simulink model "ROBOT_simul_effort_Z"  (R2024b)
settings: Solver=VariableStepAuto  StartTime=0.0  StopTime=5  RelTol=1e-3
undefined symbols (not defined in the file): a, ARRIERE_Defaut_sldprt, avant01_Defaut_sldprt, avant02_Defaut_sldprt, avant03_Defaut_sldprt, avant1_Defaut_sldprt, AXE, BASE_Defaut_sldprt, BIELLE, BIELLE_Defaut_sldprt, BRAS_Defaut_sldprt, bras_Defaut_sldprt, C_Realiste_sldprt, CABLE_Defaut_sldprt, cable_Defaut_sldprt, CACHE_Defaut_sldprt, CARTE, carte_Defaut_sldprt, CARTER, carter, CHC, CODEUR_Defaut_sldprt, cruciforme, cylindrique, deg, Drive, Fichiers, Fichiers_Matlab_sujetA, FIXATION, fixation_Defaut_sldprt, H, HEXAGONALE_Defaut_sldprt, joint_Defaut_sldprt, kg, m, M4, M4_Defaut_sldprt, manette1_Defaut_sldprt, manette2_Defaut_sldprt, MATLAB, Matlab, matlab_Defaut_sldprt, mm, modif, MOTEUR_Defaut_sldprt, N, NEZ_Defaut_sldprt, nom, palier, PARALLELOGRAMME_Defaut_sldprt, petite, plaque, rad, Ressort, Rondelle, ROTOR_Defaut_sldprt, s, SET, simple, socle_Defaut_sldprt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
libraries: sm_lib x463, fl_lib x45, nesl_utility x27, simulink x2
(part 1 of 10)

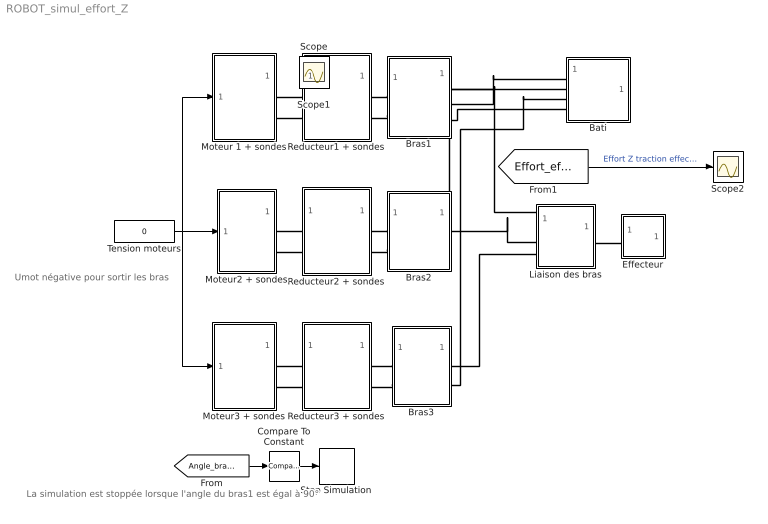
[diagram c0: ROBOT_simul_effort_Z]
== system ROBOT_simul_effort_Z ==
  note: La simulation est stoppée lorsque l'angle du bras1 est égal à 90°
  note: Umot négative pour sortir les bras
  Bati : Subsystem
  Bras1 : Subsystem
  Bras2 : Subsystem
  Bras3 : Subsystem
  Compare To Constant : simulink/Logic and Bit Operations/Compare To Constant  relop=>=  const=85  OutDataTypeStr=boolean
  Effecteur : Subsystem
  Liaison des bras : Subsystem
  Moteur 1 + sondes : Subsystem
  Moteur2 + sondes : Subsystem
  Moteur3 + sondes : Subsystem
  Reducteur1 + sondes : Subsystem
  Reducteur2 + sondes : Subsystem
  Reducteur3 + sondes : Subsystem
  Scope2 : Scope
  Stop Simulation : Stop
  Tension moteurs : Constant  Value=0
  Scope : Scope
  Scope1 : Scope
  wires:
  [Angle_bras1] -> Compare To Constant/1
  Compare To Constant/1 -> Stop Simulation/1
  Tension moteurs/1 -> Moteur2 + sondes/1(In1), Moteur 1 + sondes/1(In1), Moteur3 + sondes/1(In1)
  [Effort_effecteur] -> Scope2/1  "Effort Z traction effecteur (N)"
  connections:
  Bras3/RConn2 -- Bati/LConn3
  Bras1/LConn2 -- Reducteur1 + sondes/RConn2
  Bras2/RConn2 -- Bati/LConn2
  Moteur3 + sondes/RConn2 -- Reducteur3 + sondes/LConn2
  Bras1/RConn2 -- Bati/LConn1
  Bras1/RConn3 -- Bati/LConn4
  Liaison des bras/LConn1 -- Bras1/RConn1
  Bras3/LConn1 -- Reducteur3 + sondes/RConn1
  Moteur 1 + sondes/RConn1 -- Reducteur1 + sondes/LConn1
  Liaison des bras/LConn3 -- Bras3/RConn1
  Liaison des bras/RConn1 -- Effecteur/LConn1
  Liaison des bras/LConn2 -- Bras2/RConn1
  Moteur2 + sondes/RConn1 -- Reducteur2 + sondes/LConn1
  Bras1/LConn1 -- Reducteur1 + sondes/RConn1
  Bras3/LConn2 -- Reducteur3 + sondes/RConn2
  Moteur2 + sondes/RConn2 -- Reducteur2 + sondes/LConn2
  Bras2/LConn2 -- Reducteur2 + sondes/RConn2
  Moteur 1 + sondes/RConn2 -- Reducteur1 + sondes/LConn2
  Bras2/LConn1 -- Reducteur2 + sondes/RConn1
  Moteur3 + sondes/RConn1 -- Reducteur3 + sondes/LConn1

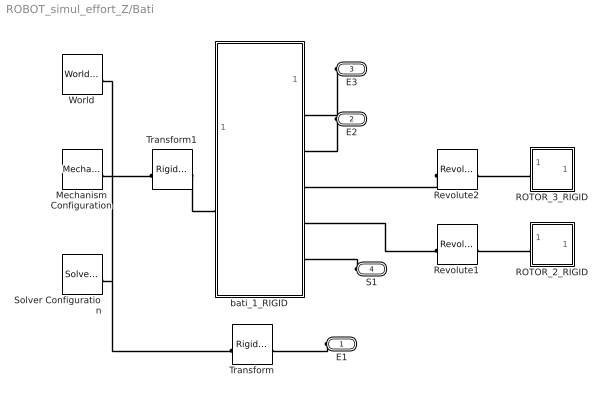
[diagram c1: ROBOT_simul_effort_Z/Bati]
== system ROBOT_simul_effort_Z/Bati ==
  Mechanism Configuration : sm_lib/Utilities/Mechanism Configuration  UniformGravity=Constant  GravityVector=[0 -9.81 0]  GravityVectorUnits=m/s^2  LinearizationDelta=0.001  JointModeTransitionNonlinearIterations=2
  ROTOR_2_RIGID : Subsystem
  ROTOR_3_RIGID : Subsystem
  Revolute1 : sm_lib/Joints/Revolute Joint  JointMode=Normal  CompositeWrenchDir=FollowerOnBase  CompositeWrenchFrame=BaseFrame  SenseConstraintForce=off  SenseConstraintTorque=off  SenseTotalForce=off  SenseTotalTorque=off  PositionTargetSpecify=on  PositionTargetPriority=Low  PositionTargetValue=-26.406351854743253  PositionTargetValueUnits=deg  VelocityTargetSpecify=off  VelocityTargetPriority=High  VelocityTargetValue=0  VelocityTargetValueUnits=deg/s  EquilibriumPosition=0  EquilibriumPositionUnits=rad  SpringStiffness=0  SpringStiffnessUnits=m*N/rad  DampingCoefficient=0  DampingCoefficientUnits=m*s*N/rad  LowerLimitSpecify=off  LowerLimitBound=-90  LowerLimitBoundUnits=deg  LowerLimitStiffness=1e4  LowerLimitStiffnessUnits=N*m/deg  LowerLimitDamping=10  LowerLimitDampingUnits=N*m/(deg/s)  LowerLimitTransitionRegionWidth=0.1  LowerLimitTransitionRegionWidthUnits=deg  UpperLimitSpecify=off  UpperLimitBound=90  UpperLimitBoundUnits=deg  UpperLimitStiffness=1e4  UpperLimitStiffnessUnits=N*m/deg  UpperLimitDamping=10  UpperLimitDampingUnits=N*m/(deg/s)  UpperLimitTransitionRegionWidth=0.1  UpperLimitTransitionRegionWidthUnits=deg  TorqueActuationMode=NoTorque  MotionActuationMode=ComputedMotion  SensePosition=off  SenseVelocity=off  SenseAcceleration=off  SenseTorqueForce=off  SenseLowerLimitTorqueForce=off  SenseUpperLimitTorqueForce=off
  Revolute2 : sm_lib/Joints/Revolute Joint  JointMode=Normal  CompositeWrenchDir=FollowerOnBase  CompositeWrenchFrame=BaseFrame  SenseConstraintForce=off  SenseConstraintTorque=off  SenseTotalForce=off  SenseTotalTorque=off  PositionTargetSpecify=on  PositionTargetPriority=Low  PositionTargetValue=-61.713604489421797  PositionTargetValueUnits=deg  VelocityTargetSpecify=off  VelocityTargetPriority=High  VelocityTargetValue=0  VelocityTargetValueUnits=deg/s  EquilibriumPosition=0  EquilibriumPositionUnits=rad  SpringStiffness=0  SpringStiffnessUnits=m*N/rad  DampingCoefficient=0  DampingCoefficientUnits=m*s*N/rad  LowerLimitSpecify=off  LowerLimitBound=-90  LowerLimitBoundUnits=deg  LowerLimitStiffness=1e4  LowerLimitStiffnessUnits=N*m/deg  LowerLimitDamping=10  LowerLimitDampingUnits=N*m/(deg/s)  LowerLimitTransitionRegionWidth=0.1  LowerLimitTransitionRegionWidthUnits=deg  UpperLimitSpecify=off  UpperLimitBound=90  UpperLimitBoundUnits=deg  UpperLimitStiffness=1e4  UpperLimitStiffnessUnits=N*m/deg  UpperLimitDamping=10  UpperLimitDampingUnits=N*m/(deg/s)  UpperLimitTransitionRegionWidth=0.1  UpperLimitTransitionRegionWidthUnits=deg  TorqueActuationMode=NoTorque  MotionActuationMode=ComputedMotion  SensePosition=off  SenseVelocity=off  SenseAcceleration=off  SenseTorqueForce=off  SenseLowerLimitTorqueForce=off  SenseUpperLimitTorqueForce=off
  Solver Configuration : nesl_utility/Solver Configuration  PhysicalDomain=network_engine_domain  SubClassName=solver  LeftPortType=input  RightPortType=generic  Tones=[]  Harmonics=[]  SimulateNoise=off  Profile=off  UseLocalSampling=off  EnableSwitchedLinearOptims=on  FrequencyDomain=off  UseCCode=off  RelTol=0.001  AbsTol=1e-06  MinStep=1e-09  ToWorkspace=off  RevertToSquareIcSolve=off  NumHomotopyIterations=100  PhasorMode=off  PhasorModeNumHarmonics=1  ConsistencySolver=NEWTON_FTOL  IndexReductionMethod=DerivativeReplacement  DoDC=off  ResidualTolerance=1e-09  ConsistencyTolSource=GLOBAL  ConsistencyAbsTol=0.001  ConsistencyRelTol=0.001  ConsistencyTolFactor=0.001  UseLocalSolver=off  LocalSolverChoice=NE_BACKWARD_EULER_ADVANCER  ResolveIndetEquations=on  FunctionEvalNumThread=1  LocalSolverSampleTime=0.001  DoFixedCost=off  MaxNonlinIter=3  MaxModeIter=2  ComputeImpulses=off  ImpulseIterations=2  LinearAlgebra=Sparse  LinearAlgebraNumThread=0  EquationFormulation=NE_TIME_EF  DelaysMemoryBudget=1024  AutomaticFiltering=on  FilteringTimeConstant=0.001  PartitionStorageMethod=AS_NEEDED  PartitionMemoryBudget=1024  PartitionMethod=FAST  MultibodyUseLocalSolver=off  MultibodyLocalSolverChoice=ODE1  MultibodyLocalSolverSampleTime=0.001
  Transform : sm_lib/Frames and Transforms/Rigid Transform  RotationMethod=ArbitraryAxis  FollAlignAxisA=+X  BaseAlignAxisA=+Y  FollAlignAxisB=+Y  BaseAlignAxisB=+Z  RotationStandardAxis=+Z  RotationAngle=2.2576709855630148  RotationAngleUnits=rad  RotationArbitraryAxis=[0.47317816576135285 0.62293756647304621 0.6229375664730461]  RotationSequenceAxes=FollowerAxes  RotationSequence=XYX  RotationSequenceAngles=[0 0 0]  RotationSequenceAnglesUnits=deg  RotationMatrix=[1 0 0; 0 1 0; 0 0 1]  Quaternion=[1 0 0 0]  TranslationMethod=Cartesian  TranslationCartesianOffset=[-50.295220189469383 24.641508789034031 0]  TranslationCartesianOffsetUnits=mm  TranslationStandardAxis=+Z  TranslationStandardOffset=0  TranslationStandardOffsetUnits=mm  TranslationROffset=0  TranslationROffsetUnits=m  TranslationThetaOffset=0  TranslationThetaOffsetUnits=deg  TranslationZOffset=0  TranslationZOffsetUnits=m
  Transform1 : sm_lib/Frames and Transforms/Rigid Transform  RotationMethod=None  FollAlignAxisA=+X  BaseAlignAxisA=+Y  FollAlignAxisB=+Y  BaseAlignAxisB=+Z  RotationStandardAxis=+Z  RotationAngle=0  RotationAngleUnits=deg  RotationArbitraryAxis=[0 0 1]  RotationSequenceAxes=FollowerAxes  RotationSequence=XYX  RotationSequenceAngles=[0 0 0]  RotationSequenceAnglesUnits=deg  RotationMatrix=[1 0 0; 0 1 0; 0 0 1]  Quaternion=[1 0 0 0]  TranslationMethod=Cartesian  TranslationCartesianOffset=[0 -115.25004756062962 -99.318100969999989]  TranslationCartesianOffsetUnits=mm  TranslationStandardAxis=+Z  TranslationStandardOffset=0  TranslationStandardOffsetUnits=mm  TranslationROffset=0  TranslationROffsetUnits=m  TranslationThetaOffset=0  TranslationThetaOffsetUnits=deg  TranslationZOffset=0  TranslationZOffsetUnits=m
  World : sm_lib/Frames and Transforms/World Frame
  bati_1_RIGID : Subsystem
  E1 : PMIOPort  Side=Left
  E2 : PMIOPort  Port=2  Side=Left
  E3 : PMIOPort  Port=3  Side=Left
  S1 : PMIOPort  Port=4  Side=Left
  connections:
  Mechanism Configuration/RConn1 -- Transform/LConn1 -- Solver Configuration/RConn1 -- World/RConn1 -- Transform1/LConn1
  ROTOR_3_RIGID/LConn1 -- Revolute2/RConn1
  Transform1/RConn1 -- bati_1_RIGID/LConn1
  Revolute2/LConn1 -- bati_1_RIGID/RConn3
  E2/RConn1 -- bati_1_RIGID/RConn2
  E1/RConn1 -- Transform/RConn1
  E3/RConn1 -- bati_1_RIGID/RConn1
  ROTOR_2_RIGID/LConn1 -- Revolute1/RConn1
  S1/RConn1 -- bati_1_RIGID/RConn5
  Revolute1/LConn1 -- bati_1_RIGID/RConn4

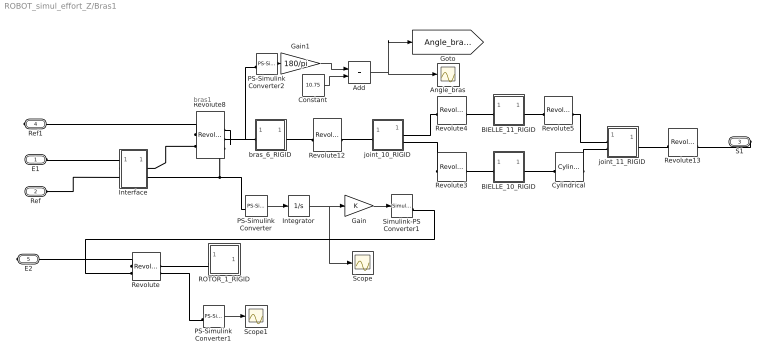
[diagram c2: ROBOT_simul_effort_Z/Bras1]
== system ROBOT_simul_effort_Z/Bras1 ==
  note: bras1
  Add : Sum
  Angle_bras : Scope
  BIELLE_10_RIGID : Subsystem
  BIELLE_11_RIGID : Subsystem
  Constant : Constant  Value=10.75
  Cylindrical : sm_lib/Joints/Cylindrical Joint  JointMode=Normal  CompositeWrenchDir=FollowerOnBase  CompositeWrenchFrame=BaseFrame  SenseConstraintForce=off  SenseConstraintTorque=off  SenseTotalForce=off  SenseTotalTorque=off  RzPositionTargetSpecify=off  RzPositionTargetPriority=High  RzPositionTargetValue=0  RzPositionTargetValueUnits=deg  RzVelocityTargetSpecify=off  RzVelocityTargetPriority=High  RzVelocityTargetValue=0  RzVelocityTargetValueUnits=deg/s  RzEquilibriumPosition=0  RzEquilibriumPositionUnits=rad  RzSpringStiffness=0  RzSpringStiffnessUnits=m*N/rad  RzDampingCoefficient=0  RzDampingCoefficientUnits=m*s*N/rad  RzLowerLimitSpecify=off  RzLowerLimitBound=-90  RzLowerLimitBoundUnits=deg  RzLowerLimitStiffness=1e4  RzLowerLimitStiffnessUnits=N*m/deg  RzLowerLimitDamping=10  RzLowerLimitDampingUnits=N*m/(deg/s)  RzLowerLimitTransitionRegionWidth=0.1  RzLowerLimitTransitionRegionWidthUnits=deg  RzUpperLimitSpecify=off  RzUpperLimitBound=90  RzUpperLimitBoundUnits=deg  RzUpperLimitStiffness=1e4  RzUpperLimitStiffnessUnits=N*m/deg  RzUpperLimitDamping=10  RzUpperLimitDampingUnits=N*m/(deg/s)  RzUpperLimitTransitionRegionWidth=0.1  RzUpperLimitTransitionRegionWidthUnits=deg  RzTorqueActuationMode=NoTorque  RzMotionActuationMode=ComputedMotion  RzSensePosition=off  RzSenseVelocity=off  RzSenseAcceleration=off  RzSenseTorqueForce=off  RzSenseLowerLimitTorqueForce=off  RzSenseUpperLimitTorqueForce=off  PzPositionTargetSpecify=off  PzPositionTargetPriority=High  PzPositionTargetValue=0  PzPositionTargetValueUnits=m  PzVelocityTargetSpecify=off  PzVelocityTargetPriority=High  PzVelocityTargetValue=0  PzVelocityTargetValueUnits=m/s  PzEquilibriumPosition=0  PzEquilibriumPositionUnits=m  PzSpringStiffness=0  PzSpringStiffnessUnits=N/m  PzDampingCoefficient=0  PzDampingCoefficientUnits=s*N/m  PzLowerLimitSpecify=off  PzLowerLimitBound=-1  PzLowerLimitBoundUnits=m  PzLowerLimitStiffness=1e6  PzLowerLimitStiffnessUnits=N/m  PzLowerLimitDamping=1e3  PzLowerLimitDampingUnits=N/(m/s)  PzLowerLimitTransitionRegionWidth=1e-4  PzLowerLimitTransitionRegionWidthUnits=m  PzUpperLimitSpecify=off  PzUpperLimitBound=1  PzUpperLimitBoundUnits=m  PzUpperLimitStiffness=1e6  PzUpperLimitStiffnessUnits=N/m  PzUpperLimitDamping=1e3  PzUpperLimitDampingUnits=N/(m/s)  PzUpperLimitTransitionRegionWidth=1e-4  PzUpperLimitTransitionRegionWidthUnits=m  PzTorqueActuationMode=NoTorque  PzMotionActuationMode=ComputedMotion  PzSensePosition=off  PzSenseVelocity=off  PzSenseAcceleration=off  PzSenseTorqueForce=off  PzSenseLowerLimitTorqueForce=off  PzSenseUpperLimitTorqueForce=off
  Gain : Gain
  Gain1 : Gain  Gain=180/pi
  Integrator : Integrator
  Interface : Subsystem
  PS-Simulink Converter : nesl_utility/PS-Simulink Converter  PhysicalDomain=network_engine_domain  SubClassName=ps_output  LeftPortType=input  RightPortType=output  PseudoPeriodic=off  Frequencies=[]  VectorFormat=1-D array  Unit=1  AffineConversion=off
  PS-Simulink Converter1 : nesl_utility/PS-Simulink Converter  PhysicalDomain=network_engine_domain  SubClassName=ps_output  LeftPortType=input  RightPortType=output  PseudoPeriodic=off  Frequencies=[]  VectorFormat=1-D array  Unit=1  AffineConversion=off
  PS-Simulink Converter2 : nesl_utility/PS-Simulink Converter  PhysicalDomain=network_engine_domain  SubClassName=ps_output  LeftPortType=input  RightPortType=output  PseudoPeriodic=off  Frequencies=[]  VectorFormat=1-D array  Unit=1  AffineConversion=off
  ROTOR_1_RIGID : Subsystem
  Revolute : sm_lib/Joints/Revolute Joint  JointMode=Normal  CompositeWrenchDir=FollowerOnBase  CompositeWrenchFrame=BaseFrame  SenseConstraintForce=off  SenseConstraintTorque=off  SenseTotalForce=off  SenseTotalTorque=off  PositionTargetSpecify=on  PositionTargetPriority=Low  PositionTargetValue=-79.560971310790379  PositionTargetValueUnits=deg  VelocityTargetSpecify=off  VelocityTargetPriority=High  VelocityTargetValue=0  VelocityTargetValueUnits=deg/s  EquilibriumPosition=0  EquilibriumPositionUnits=rad  SpringStiffness=0  SpringStiffnessUnits=m*N/rad  DampingCoefficient=0  DampingCoefficientUnits=m*s*N/rad  LowerLimitSpecify=off  LowerLimitBound=-90  LowerLimitBoundUnits=deg  LowerLimitStiffness=1e4  LowerLimitStiffnessUnits=N*m/deg  LowerLimitDamping=10  LowerLimitDampingUnits=N*m/(deg/s)  LowerLimitTransitionRegionWidth=0.1  LowerLimitTransitionRegionWidthUnits=deg  UpperLimitSpecify=off  UpperLimitBound=90  UpperLimitBoundUnits=deg  UpperLimitStiffness=1e4  UpperLimitStiffnessUnits=N*m/deg  UpperLimitDamping=10  UpperLimitDampingUnits=N*m/(deg/s)  UpperLimitTransitionRegionWidth=0.1  UpperLimitTransitionRegionWidthUnits=deg  TorqueActuationMode=ComputedTorque  MotionActuationMode=InputMotion  SensePosition=off  SenseVelocity=on  SenseAcceleration=off  SenseTorqueForce=off  SenseLowerLimitTorqueForce=off  SenseUpperLimitTorqueForce=off
  Revolute12 : sm_lib/Joints/Revolute Joint  JointMode=Normal  CompositeWrenchDir=FollowerOnBase  CompositeWrenchFrame=BaseFrame  SenseConstraintForce=off  SenseConstraintTorque=off  SenseTotalForce=off  SenseTotalTorque=off  PositionTargetSpecify=on  PositionTargetPriority=Low  PositionTargetValue=114.87234196171698  PositionTargetValueUnits=deg  VelocityTargetSpecify=off  VelocityTargetPriority=High  VelocityTargetValue=0  VelocityTargetValueUnits=deg/s  EquilibriumPosition=0  EquilibriumPositionUnits=rad  SpringStiffness=0  SpringStiffnessUnits=m*N/rad  DampingCoefficient=0  DampingCoefficientUnits=m*s*N/rad  LowerLimitSpecify=off  LowerLimitBound=-90  LowerLimitBoundUnits=deg  LowerLimitStiffness=1e4  LowerLimitStiffnessUnits=N*m/deg  LowerLimitDamping=10  LowerLimitDampingUnits=N*m/(deg/s)  LowerLimitTransitionRegionWidth=0.1  LowerLimitTransitionRegionWidthUnits=deg  UpperLimitSpecify=off  UpperLimitBound=90  UpperLimitBoundUnits=deg  UpperLimitStiffness=1e4  UpperLimitStiffnessUnits=N*m/deg  UpperLimitDamping=10  UpperLimitDampingUnits=N*m/(deg/s)  UpperLimitTransitionRegionWidth=0.1  UpperLimitTransitionRegionWidthUnits=deg  TorqueActuationMode=NoTorque  MotionActuationMode=ComputedMotion  SensePosition=off  SenseVelocity=off  SenseAcceleration=off  SenseTorqueForce=off  SenseLowerLimitTorqueForce=off  SenseUpperLimitTorqueForce=off
  Revolute13 : sm_lib/Joints/Revolute Joint  JointMode=Normal  CompositeWrenchDir=FollowerOnBase  CompositeWrenchFrame=BaseFrame  SenseConstraintForce=off  SenseConstraintTorque=off  SenseTotalForce=off  SenseTotalTorque=off  PositionTargetSpecify=off  PositionTargetPriority=High  PositionTargetValue=0  PositionTargetValueUnits=deg  VelocityTargetSpecify=off  VelocityTargetPriority=High  VelocityTargetValue=0  VelocityTargetValueUnits=deg/s  EquilibriumPosition=0  EquilibriumPositionUnits=rad  SpringStiffness=0  SpringStiffnessUnits=m*N/rad  DampingCoefficient=0  DampingCoefficientUnits=m*s*N/rad  LowerLimitSpecify=off  LowerLimitBound=-90  LowerLimitBoundUnits=deg  LowerLimitStiffness=1e4  LowerLimitStiffnessUnits=N*m/deg  LowerLimitDamping=10  LowerLimitDampingUnits=N*m/(deg/s)  LowerLimitTransitionRegionWidth=0.1  LowerLimitTransitionRegionWidthUnits=deg  UpperLimitSpecify=off  UpperLimitBound=90  UpperLimitBoundUnits=deg  UpperLimitStiffness=1e4  UpperLimitStiffnessUnits=N*m/deg  UpperLimitDamping=10  UpperLimitDampingUnits=N*m/(deg/s)  UpperLimitTransitionRegionWidth=0.1  UpperLimitTransitionRegionWidthUnits=deg  TorqueActuationMode=NoTorque  MotionActuationMode=ComputedMotion  SensePosition=off  SenseVelocity=off  SenseAcceleration=off  SenseTorqueForce=off  SenseLowerLimitTorqueForce=off  SenseUpperLimitTorqueForce=off
  Revolute3 : sm_lib/Joints/Revolute Joint  JointMode=Normal  CompositeWrenchDir=FollowerOnBase  CompositeWrenchFrame=BaseFrame  SenseConstraintForce=off  SenseConstraintTorque=off  SenseTotalForce=off  SenseTotalTorque=off  PositionTargetSpecify=on  PositionTargetPriority=Low  PositionTargetValue=-1.4448284825041595  PositionTargetValueUnits=deg  VelocityTargetSpecify=off  VelocityTargetPriority=High  VelocityTargetValue=0  VelocityTargetValueUnits=deg/s  EquilibriumPosition=0  EquilibriumPositionUnits=rad  SpringStiffness=0  SpringStiffnessUnits=m*N/rad  DampingCoefficient=0  DampingCoefficientUnits=m*s*N/rad  LowerLimitSpecify=off  LowerLimitBound=-90  LowerLimitBoundUnits=deg  LowerLimitStiffness=1e4  LowerLimitStiffnessUnits=N*m/deg  LowerLimitDamping=10  LowerLimitDampingUnits=N*m/(deg/s)  LowerLimitTransitionRegionWidth=0.1  LowerLimitTransitionRegionWidthUnits=deg  UpperLimitSpecify=off  UpperLimitBound=90  UpperLimitBoundUnits=deg  UpperLimitStiffness=1e4  UpperLimitStiffnessUnits=N*m/deg  UpperLimitDamping=10  UpperLimitDampingUnits=N*m/(deg/s)  UpperLimitTransitionRegionWidth=0.1  UpperLimitTransitionRegionWidthUnits=deg  TorqueActuationMode=NoTorque  MotionActuationMode=ComputedMotion  SensePosition=off  SenseVelocity=off  SenseAcceleration=off  SenseTorqueForce=off  SenseLowerLimitTorqueForce=off  SenseUpperLimitTorqueForce=off
  Revolute4 : sm_lib/Joints/Revolute Joint  JointMode=Normal  CompositeWrenchDir=FollowerOnBase  CompositeWrenchFrame=BaseFrame  SenseConstraintForce=off  SenseConstraintTorque=off  SenseTotalForce=off  SenseTotalTorque=off  PositionTargetSpecify=on  PositionTargetPriority=Low  PositionTargetValue=1.4448284825041535  PositionTargetValueUnits=deg  VelocityTargetSpecify=off  VelocityTargetPriority=High  VelocityTargetValue=0  VelocityTargetValueUnits=deg/s  EquilibriumPosition=0  EquilibriumPositionUnits=rad  SpringStiffness=0  SpringStiffnessUnits=m*N/rad  DampingCoefficient=0  DampingCoefficientUnits=m*s*N/rad  LowerLimitSpecify=off  LowerLimitBound=-90  LowerLimitBoundUnits=deg  LowerLimitStiffness=1e4  LowerLimitStiffnessUnits=N*m/deg  LowerLimitDamping=10  LowerLimitDampingUnits=N*m/(deg/s)  LowerLimitTransitionRegionWidth=0.1  LowerLimitTransitionRegionWidthUnits=deg  UpperLimitSpecify=off  UpperLimitBound=90  UpperLimitBoundUnits=deg  UpperLimitStiffness=1e4  UpperLimitStiffnessUnits=N*m/deg  UpperLimitDamping=10  UpperLimitDampingUnits=N*m/(deg/s)  UpperLimitTransitionRegionWidth=0.1  UpperLimitTransitionRegionWidthUnits=deg  TorqueActuationMode=NoTorque  MotionActuationMode=ComputedMotion  SensePosition=off  SenseVelocity=off  SenseAcceleration=off  SenseTorqueForce=off  SenseLowerLimitTorqueForce=off  SenseUpperLimitTorqueForce=off
  Revolute5 : sm_lib/Joints/Revolute Joint  JointMode=Normal  CompositeWrenchDir=FollowerOnBase  CompositeWrenchFrame=BaseFrame  SenseConstraintForce=off  SenseConstraintTorque=off  SenseTotalForce=off  SenseTotalTorque=off  PositionTargetSpecify=on  PositionTargetPriority=Low  PositionTargetValue=-178.55517151749589  PositionTargetValueUnits=deg  VelocityTargetSpecify=off  VelocityTargetPriority=High  VelocityTargetValue=0  VelocityTargetValueUnits=deg/s  EquilibriumPosition=0  EquilibriumPositionUnits=rad  SpringStiffness=0  SpringStiffnessUnits=m*N/rad  DampingCoefficient=0  DampingCoefficientUnits=m*s*N/rad  LowerLimitSpecify=off  LowerLimitBound=-90  LowerLimitBoundUnits=deg  LowerLimitStiffness=1e4  LowerLimitStiffnessUnits=N*m/deg  LowerLimitDamping=10  LowerLimitDampingUnits=N*m/(deg/s)  LowerLimitTransitionRegionWidth=0.1  LowerLimitTransitionRegionWidthUnits=deg  UpperLimitSpecify=off  UpperLimitBound=90  UpperLimitBoundUnits=deg  UpperLimitStiffness=1e4  UpperLimitStiffnessUnits=N*m/deg  UpperLimitDamping=10  UpperLimitDampingUnits=N*m/(deg/s)  UpperLimitTransitionRegionWidth=0.1  UpperLimitTransitionRegionWidthUnits=deg  TorqueActuationMode=NoTorque  MotionActuationMode=ComputedMotion  SensePosition=off  SenseVelocity=off  SenseAcceleration=off  SenseTorqueForce=off  SenseLowerLimitTorqueForce=off  SenseUpperLimitTorqueForce=off
  Revolute8 : sm_lib/Joints/Revolute Joint  JointMode=Normal  CompositeWrenchDir=FollowerOnBase  CompositeWrenchFrame=BaseFrame  SenseConstraintForce=off  SenseConstraintTorque=off  SenseTotalForce=off  SenseTotalTorque=off  PositionTargetSpecify=on  PositionTargetPriority=Low  PositionTargetValue=-11.877849818911594  PositionTargetValueUnits=deg  VelocityTargetSpecify=off  VelocityTargetPriority=High  VelocityTargetValue=0  VelocityTargetValueUnits=deg/s  EquilibriumPosition=0  EquilibriumPositionUnits=rad  SpringStiffness=0  SpringStiffnessUnits=m*N/rad  DampingCoefficient=0  DampingCoefficientUnits=m*s*N/rad  LowerLimitSpecify=off  LowerLimitBound=-90  LowerLimitBoundUnits=deg  LowerLimitStiffness=1e4  LowerLimitStiffnessUnits=N*m/deg  LowerLimitDamping=10  LowerLimitDampingUnits=N*m/(deg/s)  LowerLimitTransitionRegionWidth=0.1  LowerLimitTransitionRegionWidthUnits=deg  UpperLimitSpecify=off  UpperLimitBound=90  UpperLimitBoundUnits=deg  UpperLimitStiffness=1e4  UpperLimitStiffnessUnits=N*m/deg  UpperLimitDamping=10  UpperLimitDampingUnits=N*m/(deg/s)  UpperLimitTransitionRegionWidth=0.1  UpperLimitTransitionRegionWidthUnits=deg  TorqueActuationMode=InputTorque  MotionActuationMode=ComputedMotion  SensePosition=on  SenseVelocity=on  SenseAcceleration=off  SenseTorqueForce=off  SenseLowerLimitTorqueForce=off  SenseUpperLimitTorqueForce=off
  Scope : Scope
  Scope1 : Scope
  Simulink-PS Converter1 : nesl_utility/Simulink-PS Converter  PhysicalDomain=network_engine_domain  SubClassName=ps_input  LeftPortType=input  RightPortType=output  PseudoPeriodic=off  Frequencies=[]  NoiseDistribution=none  NoiseParameters=[]  Unit=1  AffineConversion=off  FilteringAndDerivatives=filter  SimscapeFilterOrder=2  InputFilterTimeConstant=1e-4  UdotUserProvided=1
  bras_6_RIGID : Subsystem
  joint_10_RIGID : Subsystem
  joint_11_RIGID : Subsystem
  E1 : PMIOPort  Side=Left
  Ref : PMIOPort  Port=2  Side=Left
  S1 : PMIOPort  Port=3  Side=Right
  Ref1 : PMIOPort  Port=4  Side=Right
  E2 : PMIOPort  Port=5  Side=Right
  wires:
  PS-Simulink Converter/1 -> Integrator/1
  Gain/1 -> Simulink-PS Converter1/1
  PS-Simulink Converter1/1 -> Scope1/1
  Integrator/1 -> Scope/1, Gain/1
  PS-Simulink Converter2/1 -> Gain1/1
  Gain1/1 -> Add/1
  Add/1 -> Angle_bras/1, [Angle_bras1]
  Constant/1 -> Add/2
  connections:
  Interface/RConn1 -- Revolute8/LConn2
  Interface/RConn2 -- Revolute8/RConn3 -- PS-Simulink Converter/LConn1
  Ref/RConn1 -- Interface/LConn2
  Interface/LConn1 -- E1/RConn1
  BIELLE_11_RIGID/LConn1 -- Revolute4/LConn1
  BIELLE_10_RIGID/RConn1 -- Cylindrical/LConn1
  Revolute4/RConn1 -- joint_10_RIGID/RConn1
  Cylindrical/RConn1 -- joint_11_RIGID/LConn2
  BIELLE_11_RIGID/RConn1 -- Revolute5/LConn1
  Revolute12/LConn1 -- bras_6_RIGID/RConn1
  Revolute12/RConn1 -- joint_10_RIGID/LConn1
  Revolute8/RConn1 -- bras_6_RIGID/LConn1
  Revolute8/LConn1 -- Ref1/RConn1
  Revolute5/RConn1 -- joint_11_RIGID/LConn1
  Revolute13/RConn1 -- joint_11_RIGID/RConn1
  S1/RConn1 -- Revolute13/LConn1
  Revolute3/RConn1 -- joint_10_RIGID/RConn2
  BIELLE_10_RIGID/LConn1 -- Revolute3/LConn1
  ROTOR_1_RIGID/LConn1 -- Revolute/RConn1
  Revolute/LConn1 -- E2/RConn1
  Revolute/LConn2 -- Simulink-PS Converter1/RConn1
  PS-Simulink Converter1/LConn1 -- Revolute/RConn2
  PS-Simulink Converter2/LConn1 -- Revolute8/RConn2

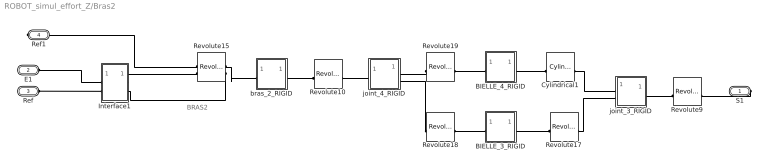
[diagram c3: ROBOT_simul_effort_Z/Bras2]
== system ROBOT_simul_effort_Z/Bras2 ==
  note: BRAS2
  BIELLE_3_RIGID : Subsystem
  BIELLE_4_RIGID : Subsystem
  Cylindrical1 : sm_lib/Joints/Cylindrical Joint  JointMode=Normal  CompositeWrenchDir=FollowerOnBase  CompositeWrenchFrame=BaseFrame  SenseConstraintForce=off  SenseConstraintTorque=off  SenseTotalForce=off  SenseTotalTorque=off  RzPositionTargetSpecify=off  RzPositionTargetPriority=High  RzPositionTargetValue=0  RzPositionTargetValueUnits=deg  RzVelocityTargetSpecify=off  RzVelocityTargetPriority=High  RzVelocityTargetValue=0  RzVelocityTargetValueUnits=deg/s  RzEquilibriumPosition=0  RzEquilibriumPositionUnits=rad  RzSpringStiffness=0  RzSpringStiffnessUnits=m*N/rad  RzDampingCoefficient=0  RzDampingCoefficientUnits=m*s*N/rad  RzLowerLimitSpecify=off  RzLowerLimitBound=-90  RzLowerLimitBoundUnits=deg  RzLowerLimitStiffness=1e4  RzLowerLimitStiffnessUnits=N*m/deg  RzLowerLimitDamping=10  RzLowerLimitDampingUnits=N*m/(deg/s)  RzLowerLimitTransitionRegionWidth=0.1  RzLowerLimitTransitionRegionWidthUnits=deg  RzUpperLimitSpecify=off  RzUpperLimitBound=90  RzUpperLimitBoundUnits=deg  RzUpperLimitStiffness=1e4  RzUpperLimitStiffnessUnits=N*m/deg  RzUpperLimitDamping=10  RzUpperLimitDampingUnits=N*m/(deg/s)  RzUpperLimitTransitionRegionWidth=0.1  RzUpperLimitTransitionRegionWidthUnits=deg  RzTorqueActuationMode=NoTorque  RzMotionActuationMode=ComputedMotion  RzSensePosition=off  RzSenseVelocity=off  RzSenseAcceleration=off  RzSenseTorqueForce=off  RzSenseLowerLimitTorqueForce=off  RzSenseUpperLimitTorqueForce=off  PzPositionTargetSpecify=off  PzPositionTargetPriority=High  PzPositionTargetValue=0  PzPositionTargetValueUnits=m  PzVelocityTargetSpecify=off  PzVelocityTargetPriority=High  PzVelocityTargetValue=0  PzVelocityTargetValueUnits=m/s  PzEquilibriumPosition=0  PzEquilibriumPositionUnits=m  PzSpringStiffness=0  PzSpringStiffnessUnits=N/m  PzDampingCoefficient=0  PzDampingCoefficientUnits=s*N/m  PzLowerLimitSpecify=off  PzLowerLimitBound=-1  PzLowerLimitBoundUnits=m  PzLowerLimitStiffness=1e6  PzLowerLimitStiffnessUnits=N/m  PzLowerLimitDamping=1e3  PzLowerLimitDampingUnits=N/(m/s)  PzLowerLimitTransitionRegionWidth=1e-4  PzLowerLimitTransitionRegionWidthUnits=m  PzUpperLimitSpecify=off  PzUpperLimitBound=1  PzUpperLimitBoundUnits=m  PzUpperLimitStiffness=1e6  PzUpperLimitStiffnessUnits=N/m  PzUpperLimitDamping=1e3  PzUpperLimitDampingUnits=N/(m/s)  PzUpperLimitTransitionRegionWidth=1e-4  PzUpperLimitTransitionRegionWidthUnits=m  PzTorqueActuationMode=NoTorque  PzMotionActuationMode=ComputedMotion  PzSensePosition=off  PzSenseVelocity=off  PzSenseAcceleration=off  PzSenseTorqueForce=off  PzSenseLowerLimitTorqueForce=off  PzSenseUpperLimitTorqueForce=off
  Interface1 : Subsystem
  Revolute10 : sm_lib/Joints/Revolute Joint  JointMode=Normal  CompositeWrenchDir=FollowerOnBase  CompositeWrenchFrame=BaseFrame  SenseConstraintForce=off  SenseConstraintTorque=off  SenseTotalForce=off  SenseTotalTorque=off  PositionTargetSpecify=on  PositionTargetPriority=Low  PositionTargetValue=114.872364906431  PositionTargetValueUnits=deg  VelocityTargetSpecify=off  VelocityTargetPriority=High  VelocityTargetValue=0  VelocityTargetValueUnits=deg/s  EquilibriumPosition=0  EquilibriumPositionUnits=rad  SpringStiffness=0  SpringStiffnessUnits=m*N/rad  DampingCoefficient=0  DampingCoefficientUnits=m*s*N/rad  LowerLimitSpecify=off  LowerLimitBound=-90  LowerLimitBoundUnits=deg  LowerLimitStiffness=1e4  LowerLimitStiffnessUnits=N*m/deg  LowerLimitDamping=10  LowerLimitDampingUnits=N*m/(deg/s)  LowerLimitTransitionRegionWidth=0.1  LowerLimitTransitionRegionWidthUnits=deg  UpperLimitSpecify=off  UpperLimitBound=90  UpperLimitBoundUnits=deg  UpperLimitStiffness=1e4  UpperLimitStiffnessUnits=N*m/deg  UpperLimitDamping=10  UpperLimitDampingUnits=N*m/(deg/s)  UpperLimitTransitionRegionWidth=0.1  UpperLimitTransitionRegionWidthUnits=deg  TorqueActuationMode=NoTorque  MotionActuationMode=ComputedMotion  SensePosition=off  SenseVelocity=off  SenseAcceleration=off  SenseTorqueForce=off  SenseLowerLimitTorqueForce=off  SenseUpperLimitTorqueForce=off
  Revolute15 : sm_lib/Joints/Revolute Joint  JointMode=Normal  CompositeWrenchDir=FollowerOnBase  CompositeWrenchFrame=BaseFrame  SenseConstraintForce=off  SenseConstraintTorque=off  SenseTotalForce=off  SenseTotalTorque=off  PositionTargetSpecify=on  PositionTargetPriority=Low  PositionTargetValue=-168.12223208512529  PositionTargetValueUnits=deg  VelocityTargetSpecify=off  VelocityTargetPriority=High  VelocityTargetValue=0  VelocityTargetValueUnits=deg/s  EquilibriumPosition=0  EquilibriumPositionUnits=rad  SpringStiffness=0  SpringStiffnessUnits=m*N/rad  DampingCoefficient=0  DampingCoefficientUnits=m*s*N/rad  LowerLimitSpecify=off  LowerLimitBound=-90  LowerLimitBoundUnits=deg  LowerLimitStiffness=1e4  LowerLimitStiffnessUnits=N*m/deg  LowerLimitDamping=10  LowerLimitDampingUnits=N*m/(deg/s)  LowerLimitTransitionRegionWidth=0.1  LowerLimitTransitionRegionWidthUnits=deg  UpperLimitSpecify=off  UpperLimitBound=90  UpperLimitBoundUnits=deg  UpperLimitStiffness=1e4  UpperLimitStiffnessUnits=N*m/deg  UpperLimitDamping=10  UpperLimitDampingUnits=N*m/(deg/s)  UpperLimitTransitionRegionWidth=0.1  UpperLimitTransitionRegionWidthUnits=deg  TorqueActuationMode=InputTorque  MotionActuationMode=ComputedMotion  SensePosition=off  SenseVelocity=on  SenseAcceleration=off  SenseTorqueForce=off  SenseLowerLimitTorqueForce=off  SenseUpperLimitTorqueForce=off
  Revolute17 : sm_lib/Joints/Revolute Joint  JointMode=Normal  CompositeWrenchDir=FollowerOnBase  CompositeWrenchFrame=BaseFrame  SenseConstraintForce=off  SenseConstraintTorque=off  SenseTotalForce=off  SenseTotalTorque=off  PositionTargetSpecify=on  PositionTargetPriority=Low  PositionTargetValue=-1.4448169961462776  PositionTargetValueUnits=deg  VelocityTargetSpecify=off  VelocityTargetPriority=High  VelocityTargetValue=0  VelocityTargetValueUnits=deg/s  EquilibriumPosition=0  EquilibriumPositionUnits=rad  SpringStiffness=0  SpringStiffnessUnits=m*N/rad  DampingCoefficient=0  DampingCoefficientUnits=m*s*N/rad  LowerLimitSpecify=off  LowerLimitBound=-90  LowerLimitBoundUnits=deg  LowerLimitStiffness=1e4  LowerLimitStiffnessUnits=N*m/deg  LowerLimitDamping=10  LowerLimitDampingUnits=N*m/(deg/s)  LowerLimitTransitionRegionWidth=0.1  LowerLimitTransitionRegionWidthUnits=deg  UpperLimitSpecify=off  UpperLimitBound=90  UpperLimitBoundUnits=deg  UpperLimitStiffness=1e4  UpperLimitStiffnessUnits=N*m/deg  UpperLimitDamping=10  UpperLimitDampingUnits=N*m/(deg/s)  UpperLimitTransitionRegionWidth=0.1  UpperLimitTransitionRegionWidthUnits=deg  TorqueActuationMode=NoTorque  MotionActuationMode=ComputedMotion  SensePosition=off  SenseVelocity=off  SenseAcceleration=off  SenseTorqueForce=off  SenseLowerLimitTorqueForce=off  SenseUpperLimitTorqueForce=off
  Revolute18 : sm_lib/Joints/Revolute Joint  JointMode=Normal  CompositeWrenchDir=FollowerOnBase  CompositeWrenchFrame=BaseFrame  SenseConstraintForce=off  SenseConstraintTorque=off  SenseTotalForce=off  SenseTotalTorque=off  PositionTargetSpecify=on  PositionTargetPriority=Low  PositionTargetValue=178.55518300385469  PositionTargetValueUnits=deg  VelocityTargetSpecify=off  VelocityTargetPriority=High  VelocityTargetValue=0  VelocityTargetValueUnits=deg/s  EquilibriumPosition=0  EquilibriumPositionUnits=rad  SpringStiffness=0  SpringStiffnessUnits=m*N/rad  DampingCoefficient=0  DampingCoefficientUnits=m*s*N/rad  LowerLimitSpecify=off  LowerLimitBound=-90  LowerLimitBoundUnits=deg  LowerLimitStiffness=1e4  LowerLimitStiffnessUnits=N*m/deg  LowerLimitDamping=10  LowerLimitDampingUnits=N*m/(deg/s)  LowerLimitTransitionRegionWidth=0.1  LowerLimitTransitionRegionWidthUnits=deg  UpperLimitSpecify=off  UpperLimitBound=90  UpperLimitBoundUnits=deg  UpperLimitStiffness=1e4  UpperLimitStiffnessUnits=N*m/deg  UpperLimitDamping=10  UpperLimitDampingUnits=N*m/(deg/s)  UpperLimitTransitionRegionWidth=0.1  UpperLimitTransitionRegionWidthUnits=deg  TorqueActuationMode=NoTorque  MotionActuationMode=ComputedMotion  SensePosition=off  SenseVelocity=off  SenseAcceleration=off  SenseTorqueForce=off  SenseLowerLimitTorqueForce=off  SenseUpperLimitTorqueForce=off
  Revolute19 : sm_lib/Joints/Revolute Joint  JointMode=Normal  CompositeWrenchDir=FollowerOnBase  CompositeWrenchFrame=BaseFrame  SenseConstraintForce=off  SenseConstraintTorque=off  SenseTotalForce=off  SenseTotalTorque=off  PositionTargetSpecify=on  PositionTargetPriority=Low  PositionTargetValue=-178.55518300385467  PositionTargetValueUnits=deg  VelocityTargetSpecify=off  VelocityTargetPriority=High  VelocityTargetValue=0  VelocityTargetValueUnits=deg/s  EquilibriumPosition=0  EquilibriumPositionUnits=rad  SpringStiffness=0  SpringStiffnessUnits=m*N/rad  DampingCoefficient=0  DampingCoefficientUnits=m*s*N/rad  LowerLimitSpecify=off  LowerLimitBound=-90  LowerLimitBoundUnits=deg  LowerLimitStiffness=1e4  LowerLimitStiffnessUnits=N*m/deg  LowerLimitDamping=10  LowerLimitDampingUnits=N*m/(deg/s)  LowerLimitTransitionRegionWidth=0.1  LowerLimitTransitionRegionWidthUnits=deg  UpperLimitSpecify=off  UpperLimitBound=90  UpperLimitBoundUnits=deg  UpperLimitStiffness=1e4  UpperLimitStiffnessUnits=N*m/deg  UpperLimitDamping=10  UpperLimitDampingUnits=N*m/(deg/s)  UpperLimitTransitionRegionWidth=0.1  UpperLimitTransitionRegionWidthUnits=deg  TorqueActuationMode=NoTorque  MotionActuationMode=ComputedMotion  SensePosition=off  SenseVelocity=off  SenseAcceleration=off  SenseTorqueForce=off  SenseLowerLimitTorqueForce=off  SenseUpperLimitTorqueForce=off
  Revolute9 : sm_lib/Joints/Revolute Joint  JointMode=Normal  CompositeWrenchDir=FollowerOnBase  CompositeWrenchFrame=BaseFrame  SenseConstraintForce=off  SenseConstraintTorque=off  SenseTotalForce=off  SenseTotalTorque=off  PositionTargetSpecify=off  PositionTargetPriority=High  PositionTargetValue=0  PositionTargetValueUnits=deg  VelocityTargetSpecify=off  VelocityTargetPriority=High  VelocityTargetValue=0  VelocityTargetValueUnits=deg/s  EquilibriumPosition=0  EquilibriumPositionUnits=rad  SpringStiffness=0  SpringStiffnessUnits=m*N/rad  DampingCoefficient=0  DampingCoefficientUnits=m*s*N/rad  LowerLimitSpecify=off  LowerLimitBound=-90  LowerLimitBoundUnits=deg  LowerLimitStiffness=1e4  LowerLimitStiffnessUnits=N*m/deg  LowerLimitDamping=10  LowerLimitDampingUnits=N*m/(deg/s)  LowerLimitTransitionRegionWidth=0.1  LowerLimitTransitionRegionWidthUnits=deg  UpperLimitSpecify=off  UpperLimitBound=90  UpperLimitBoundUnits=deg  UpperLimitStiffness=1e4  UpperLimitStiffnessUnits=N*m/deg  UpperLimitDamping=10  UpperLimitDampingUnits=N*m/(deg/s)  UpperLimitTransitionRegionWidth=0.1  UpperLimitTransitionRegionWidthUnits=deg  TorqueActuationMode=NoTorque  MotionActuationMode=ComputedMotion  SensePosition=off  SenseVelocity=off  SenseAcceleration=off  SenseTorqueForce=off  SenseLowerLimitTorqueForce=off  SenseUpperLimitTorqueForce=off
  bras_2_RIGID : Subsystem
  joint_3_RIGID : Subsystem
  joint_4_RIGID : Subsystem
  S1 : PMIOPort  Side=Right
  E1 : PMIOPort  Port=2  Side=Left
  Ref : PMIOPort  Port=3  Side=Left
  Ref1 : PMIOPort  Port=4  Side=Right
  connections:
  Interface1/RConn2 -- Revolute15/RConn2
  Interface1/RConn1 -- Revolute15/LConn2
  Interface1/LConn1 -- E1/RConn1
  Interface1/LConn2 -- Ref/RConn1
  BIELLE_3_RIGID/LConn1 -- Revolute17/RConn1
  Cylindrical1/LConn1 -- joint_3_RIGID/LConn1
  Revolute15/RConn1 -- bras_2_RIGID/LConn1
  Revolute10/RConn1 -- joint_4_RIGID/LConn1
  Revolute17/LConn1 -- joint_3_RIGID/LConn2
  Revolute10/LConn1 -- bras_2_RIGID/RConn1
  S1/RConn1 -- Revolute9/RConn1
  Revolute9/LConn1 -- joint_3_RIGID/RConn1
  BIELLE_3_RIGID/RConn1 -- Revolute18/LConn1
  Revolute15/LConn1 -- Ref1/RConn1
  Revolute18/RConn1 -- joint_4_RIGID/RConn2
  BIELLE_4_RIGID/LConn1 -- Cylindrical1/RConn1
  Revolute19/RConn1 -- joint_4_RIGID/RConn1
  BIELLE_4_RIGID/RConn1 -- Revolute19/LConn1

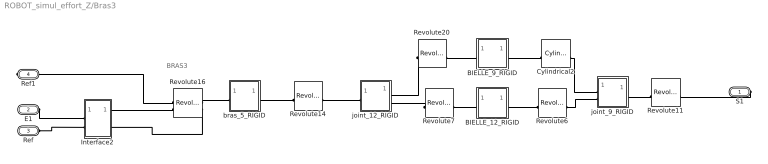
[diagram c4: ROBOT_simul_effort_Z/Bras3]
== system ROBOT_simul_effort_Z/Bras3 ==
  note: BRAS3
  BIELLE_12_RIGID : Subsystem
  BIELLE_9_RIGID : Subsystem
  Cylindrical2 : sm_lib/Joints/Cylindrical Joint  JointMode=Normal  CompositeWrenchDir=FollowerOnBase  CompositeWrenchFrame=BaseFrame  SenseConstraintForce=off  SenseConstraintTorque=off  SenseTotalForce=off  SenseTotalTorque=off  RzPositionTargetSpecify=off  RzPositionTargetPriority=High  RzPositionTargetValue=0  RzPositionTargetValueUnits=deg  RzVelocityTargetSpecify=off  RzVelocityTargetPriority=High  RzVelocityTargetValue=0  RzVelocityTargetValueUnits=deg/s  RzEquilibriumPosition=0  RzEquilibriumPositionUnits=rad  RzSpringStiffness=0  RzSpringStiffnessUnits=m*N/rad  RzDampingCoefficient=0  RzDampingCoefficientUnits=m*s*N/rad  RzLowerLimitSpecify=off  RzLowerLimitBound=-90  RzLowerLimitBoundUnits=deg  RzLowerLimitStiffness=1e4  RzLowerLimitStiffnessUnits=N*m/deg  RzLowerLimitDamping=10  RzLowerLimitDampingUnits=N*m/(deg/s)  RzLowerLimitTransitionRegionWidth=0.1  RzLowerLimitTransitionRegionWidthUnits=deg  RzUpperLimitSpecify=off  RzUpperLimitBound=90  RzUpperLimitBoundUnits=deg  RzUpperLimitStiffness=1e4  RzUpperLimitStiffnessUnits=N*m/deg  RzUpperLimitDamping=10  RzUpperLimitDampingUnits=N*m/(deg/s)  RzUpperLimitTransitionRegionWidth=0.1  RzUpperLimitTransitionRegionWidthUnits=deg  RzTorqueActuationMode=NoTorque  RzMotionActuationMode=ComputedMotion  RzSensePosition=off  RzSenseVelocity=off  RzSenseAcceleration=off  RzSenseTorqueForce=off  RzSenseLowerLimitTorqueForce=off  RzSenseUpperLimitTorqueForce=off  PzPositionTargetSpecify=off  PzPositionTargetPriority=High  PzPositionTargetValue=0  PzPositionTargetValueUnits=m  PzVelocityTargetSpecify=off  PzVelocityTargetPriority=High  PzVelocityTargetValue=0  PzVelocityTargetValueUnits=m/s  PzEquilibriumPosition=0  PzEquilibriumPositionUnits=m  PzSpringStiffness=0  PzSpringStiffnessUnits=N/m  PzDampingCoefficient=0  PzDampingCoefficientUnits=s*N/m  PzLowerLimitSpecify=off  PzLowerLimitBound=-1  PzLowerLimitBoundUnits=m  PzLowerLimitStiffness=1e6  PzLowerLimitStiffnessUnits=N/m  PzLowerLimitDamping=1e3  PzLowerLimitDampingUnits=N/(m/s)  PzLowerLimitTransitionRegionWidth=1e-4  PzLowerLimitTransitionRegionWidthUnits=m  PzUpperLimitSpecify=off  PzUpperLimitBound=1  PzUpperLimitBoundUnits=m  PzUpperLimitStiffness=1e6  PzUpperLimitStiffnessUnits=N/m  PzUpperLimitDamping=1e3  PzUpperLimitDampingUnits=N/(m/s)  PzUpperLimitTransitionRegionWidth=1e-4  PzUpperLimitTransitionRegionWidthUnits=m  PzTorqueActuationMode=NoTorque  PzMotionActuationMode=ComputedMotion  PzSensePosition=off  PzSenseVelocity=off  PzSenseAcceleration=off  PzSenseTorqueForce=off  PzSenseLowerLimitTorqueForce=off  PzSenseUpperLimitTorqueForce=off
  Interface2 : Subsystem
  Revolute11 : sm_lib/Joints/Revolute Joint  JointMode=Normal  CompositeWrenchDir=FollowerOnBase  CompositeWrenchFrame=BaseFrame  SenseConstraintForce=off  SenseConstraintTorque=off  SenseTotalForce=off  SenseTotalTorque=off  PositionTargetSpecify=on  PositionTargetPriority=Low  PositionTargetValue=36.757042846011267  PositionTargetValueUnits=deg  VelocityTargetSpecify=off  VelocityTargetPriority=High  VelocityTargetValue=0  VelocityTargetValueUnits=deg/s  EquilibriumPosition=0  EquilibriumPositionUnits=rad  SpringStiffness=0  SpringStiffnessUnits=m*N/rad  DampingCoefficient=0  DampingCoefficientUnits=m*s*N/rad  LowerLimitSpecify=off  LowerLimitBound=-90  LowerLimitBoundUnits=deg  LowerLimitStiffness=1e4  LowerLimitStiffnessUnits=N*m/deg  LowerLimitDamping=10  LowerLimitDampingUnits=N*m/(deg/s)  LowerLimitTransitionRegionWidth=0.1  LowerLimitTransitionRegionWidthUnits=deg  UpperLimitSpecify=off  UpperLimitBound=90  UpperLimitBoundUnits=deg  UpperLimitStiffness=1e4  UpperLimitStiffnessUnits=N*m/deg  UpperLimitDamping=10  UpperLimitDampingUnits=N*m/(deg/s)  UpperLimitTransitionRegionWidth=0.1  UpperLimitTransitionRegionWidthUnits=deg  TorqueActuationMode=NoTorque  MotionActuationMode=ComputedMotion  SensePosition=off  SenseVelocity=off  SenseAcceleration=off  SenseTorqueForce=off  SenseLowerLimitTorqueForce=off  SenseUpperLimitTorqueForce=off
  Revolute14 : sm_lib/Joints/Revolute Joint  JointMode=Normal  CompositeWrenchDir=FollowerOnBase  CompositeWrenchFrame=BaseFrame  SenseConstraintForce=off  SenseConstraintTorque=off  SenseTotalForce=off  SenseTotalTorque=off  PositionTargetSpecify=on  PositionTargetPriority=Low  PositionTargetValue=114.86123956506862  PositionTargetValueUnits=deg  VelocityTargetSpecify=off  VelocityTargetPriority=High  VelocityTargetValue=0  VelocityTargetValueUnits=deg/s  EquilibriumPosition=0  EquilibriumPositionUnits=rad  SpringStiffness=0  SpringStiffnessUnits=m*N/rad  DampingCoefficient=0  DampingCoefficientUnits=m*s*N/rad  LowerLimitSpecify=off  LowerLimitBound=-90  LowerLimitBoundUnits=deg  LowerLimitStiffness=1e4  LowerLimitStiffnessUnits=N*m/deg  LowerLimitDamping=10  LowerLimitDampingUnits=N*m/(deg/s)  LowerLimitTransitionRegionWidth=0.1  LowerLimitTransitionRegionWidthUnits=deg  UpperLimitSpecify=off  UpperLimitBound=90  UpperLimitBoundUnits=deg  UpperLimitStiffness=1e4  UpperLimitStiffnessUnits=N*m/deg  UpperLimitDamping=10  UpperLimitDampingUnits=N*m/(deg/s)  UpperLimitTransitionRegionWidth=0.1  UpperLimitTransitionRegionWidthUnits=deg  TorqueActuationMode=NoTorque  MotionActuationMode=ComputedMotion  SensePosition=off  SenseVelocity=off  SenseAcceleration=off  SenseTorqueForce=off  SenseLowerLimitTorqueForce=off  SenseUpperLimitTorqueForce=off
  Revolute16 : sm_lib/Joints/Revolute Joint  JointMode=Normal  CompositeWrenchDir=FollowerOnBase  CompositeWrenchFrame=BaseFrame  SenseConstraintForce=off  SenseConstraintTorque=off  SenseTotalForce=off  SenseTotalTorque=off  PositionTargetSpecify=on  PositionTargetPriority=Low  PositionTargetValue=101.89580328094226  PositionTargetValueUnits=deg  VelocityTargetSpecify=off  VelocityTargetPriority=High  VelocityTargetValue=0  VelocityTargetValueUnits=deg/s  EquilibriumPosition=0  EquilibriumPositionUnits=rad  SpringStiffness=0  SpringStiffnessUnits=m*N/rad  DampingCoefficient=0  DampingCoefficientUnits=m*s*N/rad  LowerLimitSpecify=off  LowerLimitBound=-90  LowerLimitBoundUnits=deg  LowerLimitStiffness=1e4  LowerLimitStiffnessUnits=N*m/deg  LowerLimitDamping=10  LowerLimitDampingUnits=N*m/(deg/s)  LowerLimitTransitionRegionWidth=0.1  LowerLimitTransitionRegionWidthUnits=deg  UpperLimitSpecify=off  UpperLimitBound=90  UpperLimitBoundUnits=deg  UpperLimitStiffness=1e4  UpperLimitStiffnessUnits=N*m/deg  UpperLimitDamping=10  UpperLimitDampingUnits=N*m/(deg/s)  UpperLimitTransitionRegionWidth=0.1  UpperLimitTransitionRegionWidthUnits=deg  TorqueActuationMode=InputTorque  MotionActuationMode=ComputedMotion  SensePosition=off  SenseVelocity=on  SenseAcceleration=off  SenseTorqueForce=off  SenseLowerLimitTorqueForce=off  SenseUpperLimitTorqueForce=off
  Revolute20 : sm_lib/Joints/Revolute Joint  JointMode=Normal  CompositeWrenchDir=FollowerOnBase  CompositeWrenchFrame=BaseFrame  SenseConstraintForce=off  SenseConstraintTorque=off  SenseTotalForce=off  SenseTotalTorque=off  PositionTargetSpecify=on  PositionTargetPriority=Low  PositionTargetValue=-178.83470303505044  PositionTargetValueUnits=deg  VelocityTargetSpecify=off  VelocityTargetPriority=High  VelocityTargetValue=0  VelocityTargetValueUnits=deg/s  EquilibriumPosition=0  EquilibriumPositionUnits=rad  SpringStiffness=0  SpringStiffnessUnits=m*N/rad  DampingCoefficient=0  DampingCoefficientUnits=m*s*N/rad  LowerLimitSpecify=off  LowerLimitBound=-90  LowerLimitBoundUnits=deg  LowerLimitStiffness=1e4  LowerLimitStiffnessUnits=N*m/deg  LowerLimitDamping=10  LowerLimitDampingUnits=N*m/(deg/s)  LowerLimitTransitionRegionWidth=0.1  LowerLimitTransitionRegionWidthUnits=deg  UpperLimitSpecify=off  UpperLimitBound=90  UpperLimitBoundUnits=deg  UpperLimitStiffness=1e4  UpperLimitStiffnessUnits=N*m/deg  UpperLimitDamping=10  UpperLimitDampingUnits=N*m/(deg/s)  UpperLimitTransitionRegionWidth=0.1  UpperLimitTransitionRegionWidthUnits=deg  TorqueActuationMode=NoTorque  MotionActuationMode=ComputedMotion  SensePosition=off  SenseVelocity=off  SenseAcceleration=off  SenseTorqueForce=off  SenseLowerLimitTorqueForce=off  SenseUpperLimitTorqueForce=off
  Revolute6 : sm_lib/Joints/Revolute Joint  JointMode=Normal  CompositeWrenchDir=FollowerOnBase  CompositeWrenchFrame=BaseFrame  SenseConstraintForce=off  SenseConstraintTorque=off  SenseTotalForce=off  SenseTotalTorque=off  PositionTargetSpecify=on  PositionTargetPriority=Low  PositionTargetValue=-178.83470303504936  PositionTargetValueUnits=deg  VelocityTargetSpecify=off  VelocityTargetPriority=High  VelocityTargetValue=0  VelocityTargetValueUnits=deg/s  EquilibriumPosition=0  EquilibriumPositionUnits=rad  SpringStiffness=0  SpringStiffnessUnits=m*N/rad  DampingCoefficient=0  DampingCoefficientUnits=m*s*N/rad  LowerLimitSpecify=off  LowerLimitBound=-90  LowerLimitBoundUnits=deg  LowerLimitStiffness=1e4  LowerLimitStiffnessUnits=N*m/deg  LowerLimitDamping=10  LowerLimitDampingUnits=N*m/(deg/s)  LowerLimitTransitionRegionWidth=0.1  LowerLimitTransitionRegionWidthUnits=deg  UpperLimitSpecify=off  UpperLimitBound=90  UpperLimitBoundUnits=deg  UpperLimitStiffness=1e4  UpperLimitStiffnessUnits=N*m/deg  UpperLimitDamping=10  UpperLimitDampingUnits=N*m/(deg/s)  UpperLimitTransitionRegionWidth=0.1  UpperLimitTransitionRegionWidthUnits=deg  TorqueActuationMode=NoTorque  MotionActuationMode=ComputedMotion  SensePosition=off  SenseVelocity=off  SenseAcceleration=off  SenseTorqueForce=off  SenseLowerLimitTorqueForce=off  SenseUpperLimitTorqueForce=off
  Revolute7 : sm_lib/Joints/Revolute Joint  JointMode=Normal  CompositeWrenchDir=FollowerOnBase  CompositeWrenchFrame=BaseFrame  SenseConstraintForce=off  SenseConstraintTorque=off  SenseTotalForce=off  SenseTotalTorque=off  PositionTargetSpecify=on  PositionTargetPriority=Low  PositionTargetValue=1.1652969649496245  PositionTargetValueUnits=deg  VelocityTargetSpecify=off  VelocityTargetPriority=High  VelocityTargetValue=0  VelocityTargetValueUnits=deg/s  EquilibriumPosition=0  EquilibriumPositionUnits=rad  SpringStiffness=0  SpringStiffnessUnits=m*N/rad  DampingCoefficient=0  DampingCoefficientUnits=m*s*N/rad  LowerLimitSpecify=off  LowerLimitBound=-90  LowerLimitBoundUnits=deg  LowerLimitStiffness=1e4  LowerLimitStiffnessUnits=N*m/deg  LowerLimitDamping=10  LowerLimitDampingUnits=N*m/(deg/s)  LowerLimitTransitionRegionWidth=0.1  LowerLimitTransitionRegionWidthUnits=deg  UpperLimitSpecify=off  UpperLimitBound=90  UpperLimitBoundUnits=deg  UpperLimitStiffness=1e4  UpperLimitStiffnessUnits=N*m/deg  UpperLimitDamping=10  UpperLimitDampingUnits=N*m/(deg/s)  UpperLimitTransitionRegionWidth=0.1  UpperLimitTransitionRegionWidthUnits=deg  TorqueActuationMode=NoTorque  MotionActuationMode=ComputedMotion  SensePosition=off  SenseVelocity=off  SenseAcceleration=off  SenseTorqueForce=off  SenseLowerLimitTorqueForce=off  SenseUpperLimitTorqueForce=off
  bras_5_RIGID : Subsystem
  joint_12_RIGID : Subsystem
  joint_9_RIGID : Subsystem
  S1 : PMIOPort  Side=Right
  E1 : PMIOPort  Port=2  Side=Left
  Ref : PMIOPort  Port=3  Side=Left
  Ref1 : PMIOPort  Port=4  Side=Right
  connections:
  Interface2/RConn2 -- Revolute16/RConn2
  Interface2/RConn1 -- Revolute16/LConn2
  E1/RConn1 -- Interface2/LConn1
  Ref/RConn1 -- Interface2/LConn2
  Revolute11/RConn1 -- joint_9_RIGID/RConn1
  Revolute7/RConn1 -- joint_12_RIGID/RConn2
  Revolute14/RConn1 -- joint_12_RIGID/LConn1
  S1/RConn1 -- Revolute11/LConn1
  Revolute14/LConn1 -- bras_5_RIGID/RConn1
  Revolute16/LConn1 -- Ref1/RConn1
  Revolute16/RConn1 -- bras_5_RIGID/LConn1
  Revolute6/LConn1 -- BIELLE_12_RIGID/RConn1
  BIELLE_12_RIGID/LConn1 -- Revolute7/LConn1
  Revolute6/RConn1 -- joint_9_RIGID/LConn2
  Revolute20/RConn1 -- joint_12_RIGID/RConn1
  BIELLE_9_RIGID/LConn1 -- Revolute20/LConn1
  BIELLE_9_RIGID/RConn1 -- Cylindrical2/LConn1
  Cylindrical2/RConn1 -- joint_9_RIGID/LConn1
